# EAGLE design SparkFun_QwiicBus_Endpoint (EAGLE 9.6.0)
ABBREV: hb1; PROJECT: Heading Board
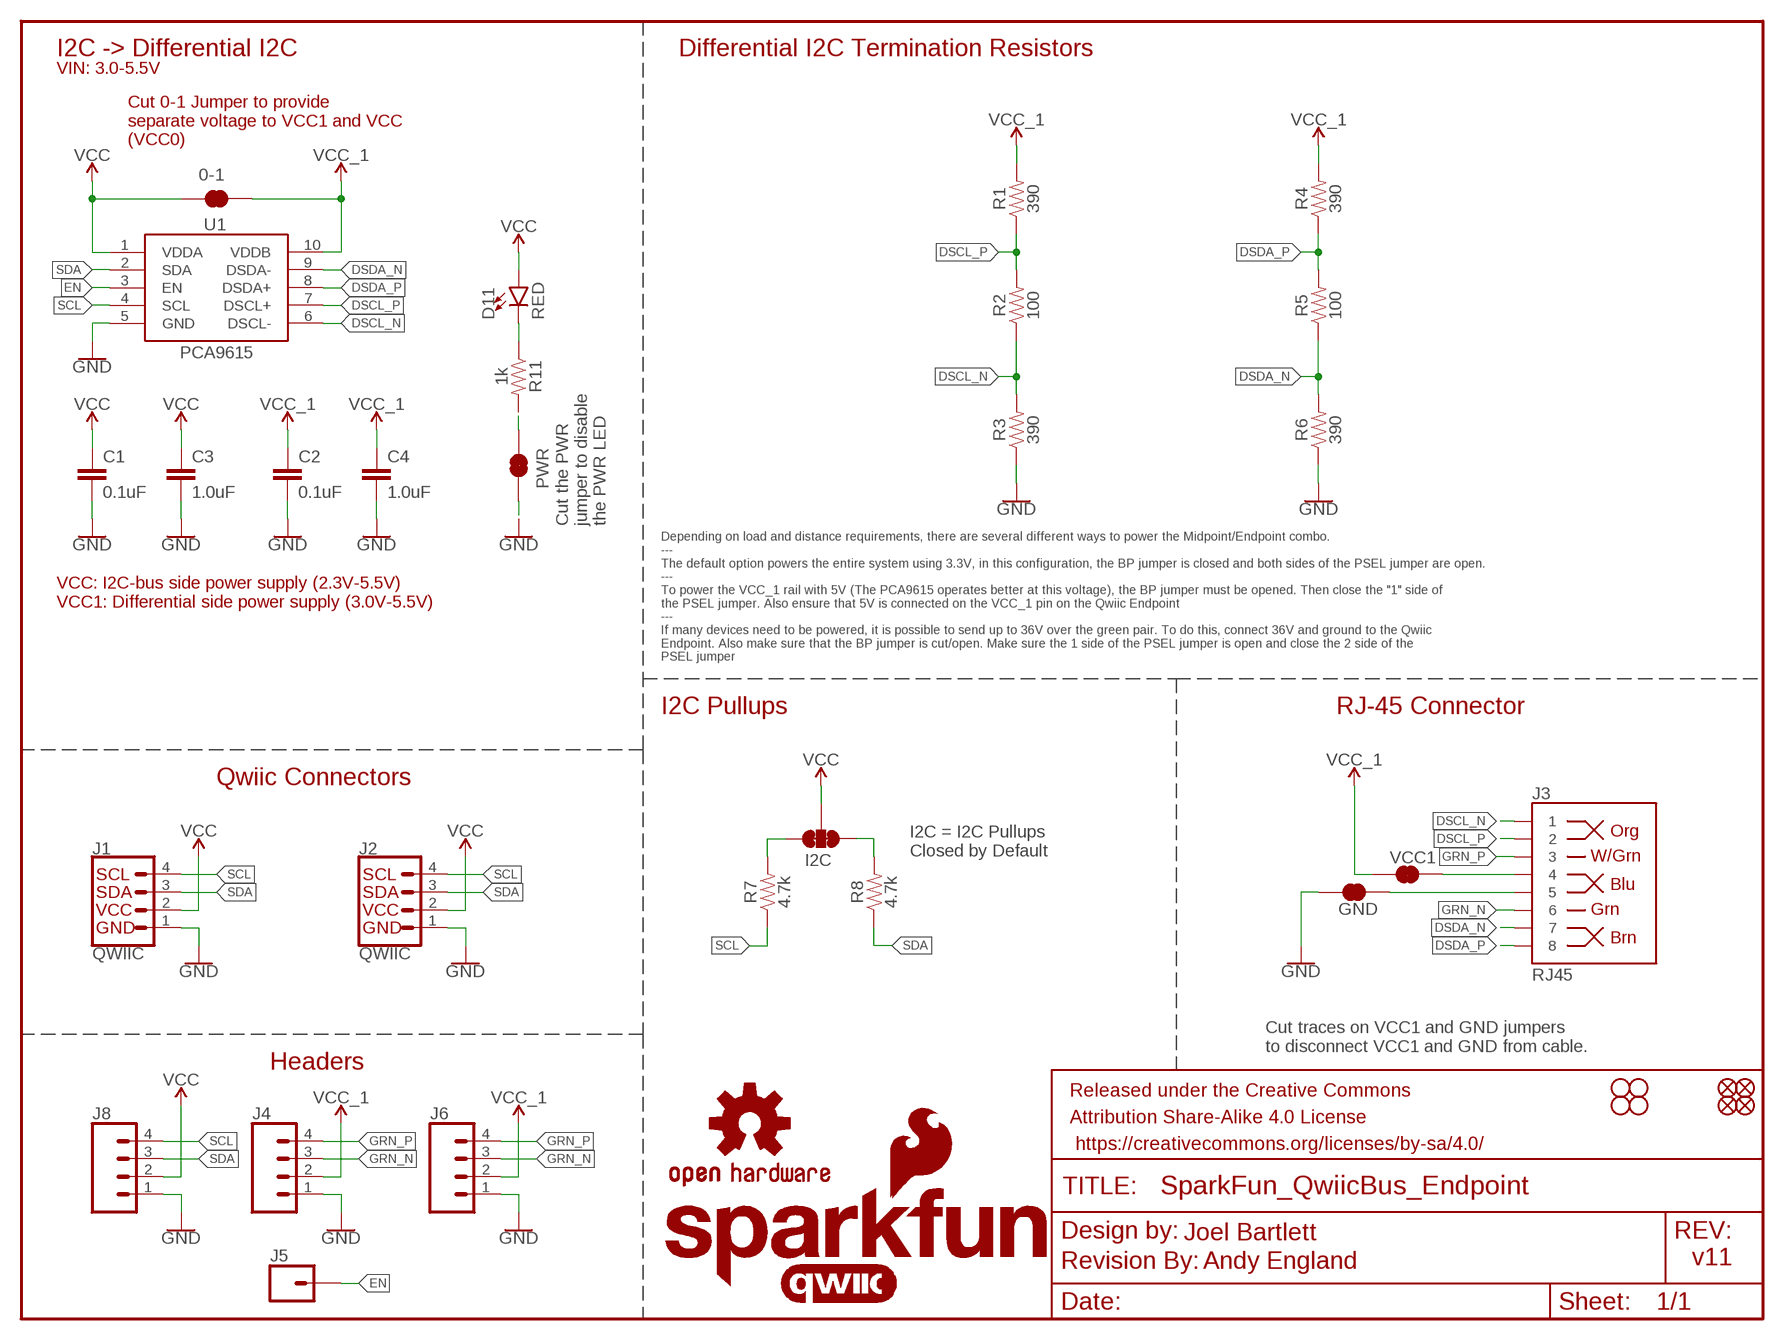
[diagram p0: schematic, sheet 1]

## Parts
0-1  JUMPER-SMT_2_NC_TRACE_SILK  [SMT-JUMPER_2_NC_TRACE_SILK]
C1  0.1uF  0.1UF-0603-25V-(+80/-20%)  [0603]
C2  0.1uF  0.1UF-0603-25V-(+80/-20%)  [0603]
C3  1.0uF  1.0UF-0603-16V-10%  [0603]
C4  1.0uF  1.0UF-0603-16V-10%  [0603]
D11  RED  LED-RED0603  [LED-0603]
FD1  FIDUCIALUFIDUCIAL  [FIDUCIAL-MICRO]
FD2  FIDUCIALUFIDUCIAL  [FIDUCIAL-MICRO]
FD3  FIDUCIALUFIDUCIAL  [FIDUCIAL-MICRO]
FD4  FIDUCIALUFIDUCIAL  [FIDUCIAL-MICRO]
FRAME1  FRAME-LETTER  [CREATIVE_COMMONS]
GND  JUMPER-SMT_2_NC_TRACE_SILK  [SMT-JUMPER_2_NC_TRACE_SILK]
H1  STAND-OFF  [STAND-OFF]
H2  STAND-OFF  [STAND-OFF]
H3  STAND-OFF  [STAND-OFF]
H4  STAND-OFF  [STAND-OFF]
I2C  JUMPER-SMT_3_2-NC_TRACE_SILK  [SMT-JUMPER_3_2-NC_TRACE_SILK]
J1  QWIIC  QWIIC_CONNECTORJS-1MM  [JST04_1MM_RA]
J2  QWIIC  QWIIC_CONNECTORJS-1MM  [JST04_1MM_RA]
J3  RJ45  RJ45-8  [RJ45-8]
J4  CONN_041X04_NO_SILK  [1X04_NO_SILK]
J5  CONN_01PTH_NO_SILK_YES_STOP  [1X01_NO_SILK]
J6  CONN_041X04_NO_SILK  [1X04_NO_SILK]
J8  CONN_041X04_NO_SILK  [1X04_NO_SILK]
LOGO1  OSHW-LOGOM  [OSHW-LOGO-M]
LOGO2  REVISION  [REVISION]
LOGO3  QWIIC_LOGO_4MM  [QWIIC_4MM]
LOGO4  SFE_LOGO_NAME_FLAME.1_INCH  [SFE_LOGO_NAME_FLAME_.1]
LOGO5  SFE_LOGO_FLAME.1_INCH  [SFE_LOGO_FLAME_.1]
PWR  JUMPER-SMT_2_NC_TRACE_SILK  [SMT-JUMPER_2_NC_TRACE_SILK]
R1  390  390OHM-0603-1/10W-1%  [0603]
R2  100  100OHM-0603-1/10W-1%  [0603]
R3  390  390OHM-0603-1/10W-1%  [0603]
R4  390  390OHM-0603-1/10W-1%  [0603]
R5  100  100OHM-0603-1/10W-1%  [0603]
R6  390  390OHM-0603-1/10W-1%  [0603]
R7  4.7k  4.7KOHM-0603-1/10W-1%  [0603]
R8  4.7k  4.7KOHM-0603-1/10W-1%  [0603]
R11  1k  1KOHM-0603-1/10W-1%  [0603]
U1  PCA9615  [TSSOP10]
VCC1  JUMPER-SMT_2_NC_TRACE_SILK  [SMT-JUMPER_2_NC_TRACE_SILK]

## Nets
DSCL_N: J3.1 R2.1 R3.2 U1.6(DSCL-)
DSCL_P: J3.2 R1.1 R2.2 U1.7(DSCL+)
DSDA_N: J3.7 R5.1 R6.2 U1.9(DSDA-)
DSDA_P: J3.8 R4.1 R5.2 U1.8(DSDA+)
EN: J5.1 U1.3(EN)
GND: C1.2 C2.2 C3.2 C4.2 GND.1 J1.1 J2.1 J4.1 J6.1 J8.1 PWR.1 R3.1 R6.1 U1.5(GND)
GRN_N: J3.6 J4.3 J6.3
GRN_P: J3.3 J4.4 J6.4
N$1: J3.4 VCC1.2
N$2: GND.2 J3.5
N$3: I2C.1 R8.2
N$4: I2C.3 R7.2
N$13: D11.C R11.1
N$14: PWR.2 R11.2
SCL: J1.4 J2.4 J8.4 R7.1 U1.4(SCL)
SDA: J1.3 J2.3 J8.3 R8.1 U1.2(SDA)
VCC: 0-1.2 C1.1 C3.1 D11.A I2C.2 J1.2 J2.2 J8.2 U1.1(VDDA)
VCC_1: 0-1.1 C2.1 C4.1 J4.2 J6.2 R1.2 R4.2 U1.10(VDDB) VCC1.1

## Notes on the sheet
- I2C -> Differential I2C | Differential I2C Termination Resistors
- VIN: 3.0-5.5V
- Cut 0-1 Jumper to provide
  separate voltage to VCC1 and VCC
  (VCC0)
- Cut the PWR 
  jumper to disable
  the PWR LED
- VCC: I2C-bus side power supply (2.3V-5.5V)
  VCC1: Differential side power supply (3.0V-5.5V)
- Depending on load and distance requirements, there are several different ways to power the Midpoint/Endpoint combo. 
  ---
  The default option powers the entire system using 3.3V, in this configuration, the BP jumper is closed and both sides of the PSEL jumper are open.
  ---
  To power the VCC_1 rail with 5V (The PCA9615 operates better at this voltage), the BP jumper must be opened. Then close the "1" side of 
  the PSEL jumper. Also ensure that 5V is connected on the VCC_1 pin on the Qwiic Endpoint
  ---
  If many devices need to be powered, it is possible to send up to 36V over the green pair. To do this, connect 36V and ground to the Qwiic 
  Endpoint. Also make sure that the BP jumper is cut/open. Make sure the 1 side of the PSEL jumper is open and close the 2 side of the
  PSEL jumper
- I2C Pullups | RJ-45 Connector
- Qwiic Connectors
- I2C = I2C Pullups
  Closed by Default
- Cut traces on VCC1 and GND jumpers 
  to disconnect VCC1 and GND from cable.
- Headers
- Joel Bartlett
- Andy England | v11

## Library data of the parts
0-1 GND PWR VCC1 = SparkFun-Jumpers:JUMPER-SMT_2_NC_TRACE: Normally closed trace jumper
C1 C2 = SparkFun-Capacitors:0.1UF: 0.1µF ceramic capacitors; PROD_ID: CAP-00810
C3 C4 = SparkFun-Capacitors:1.0UF: 1µF ceramic capacitors; PROD_ID: CAP-00868
D11 = SparkFun-LED:LED-RED: Red SMD LED; PROD_ID: DIO-00819
FD1-FD4 = SparkFun-Aesthetics:FIDUCIAL: Fiducial Alignment Points
FRAME1 = SparkFun-Aesthetics:FRAME-LETTER: Schematic Frame - Letter
H1-H4 = SparkFun-Hardware:STAND-OFF: Stand Off
I2C = SparkFun-Jumpers:JUMPER-SMT_3_2-NC_TRACE: Normally closed trace jumper (2 of 2 connections) This jumper has a trace between all three pads so they are normally closed (NC). Use a razor knife to open the connection(s). For best results follow the IPC guidelines for cutting traces: Cutout at least 0.063 mm (0.005 in). Remove all loose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
J1 J2 = SparkFun-Connectors:QWIIC_CONNECTOR: SparkFun I2C Standard Qwiic Connector An SMD 1mm pitch JST connector makes it easy and quick (get it? Qwiic?) to connect I2C devices to each other. The Qwiic system enables fast and solderless connection between popular platforms and various sensors and actuators. We carry 200mm, 100mm, 50mm, and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; PROD_ID: CONN-13694; VALUE: QWIIC_RIGHT_ANGLE
J3 = SparkFun-Connectors:RJ45-8: RJ45 Jack - 8 pin Simple RJ45, 8-pin connection. Commonly used for Cat5, Cat5e, and Cat6 Ethernet cables. Here is the connector we sell at SparkFun: RJ45 8-Pin Connector (PRT-00643) Datasheet It is used on this SparkFun product: SparkFun RJ45 Breakout (BOB-00716) Note, you may also be interested in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; PROD_ID: CONN-08506; SF_ID: PRT-00643
J4 J6 J8 = SparkFun-Connectors:CONN_04: Multi connection point. Often used as Generic Header-pin footprint for 0.1 inch spaced/style header connections On any of the 0.1 inch spaced packages, you can populate with these: Break Away Headers - Straight (PRT-00116) Break Away Male Headers - Right Angle (PRT-00553) Female Headers (PRT-00115)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; PROD_ID: CONN-09696
J5 = SparkFun-Connectors:CONN_01: Single connection point. Often used as Generic Header-pin footprint for 0.1 inch spaced/style header connections
LOGO1 = SparkFun-Aesthetics:OSHW-LOGO: Open-Source Hardware (OSHW) Logo
LOGO2 = SparkFun-Aesthetics:REVISION: "Revision By" Text
LOGO3 = SparkFun-Aesthetics:QWIIC_LOGO: Qwiic Logos for placement on schematic and PCB. The 5.5mm silk logo is best for placing next to Qwiic connector.
LOGO4 = SparkFun-Aesthetics:SFE_LOGO_NAME_FLAME: SparkFun Font Logo w/ Flame
LOGO5 = SparkFun-Aesthetics:SFE_LOGO_FLAME: SparkFun Flame Logo
R1 R3 R4 R6 = SparkFun-Resistors:390OHM: 390Ω resistor; PROD_ID: RES-07864
R2 R5 = SparkFun-Resistors:100OHM: 100Ω resistor; PROD_ID: RES-07863
R7 R8 = SparkFun-Resistors:4.7KOHM: 4.7kΩ resistor; PROD_ID: RES-07857
R11 = SparkFun-Resistors:1KOHM: 1kΩ resistor; PROD_ID: RES-07856
U1 = SparkFun-IC-Comms:PCA9615: Differential I2C Bus Buffer Datasheet; PROD_ID: IC-13899

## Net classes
0 default: width 0.203 mm
1 power: width 0.381 mm, clearance 0.254 mm

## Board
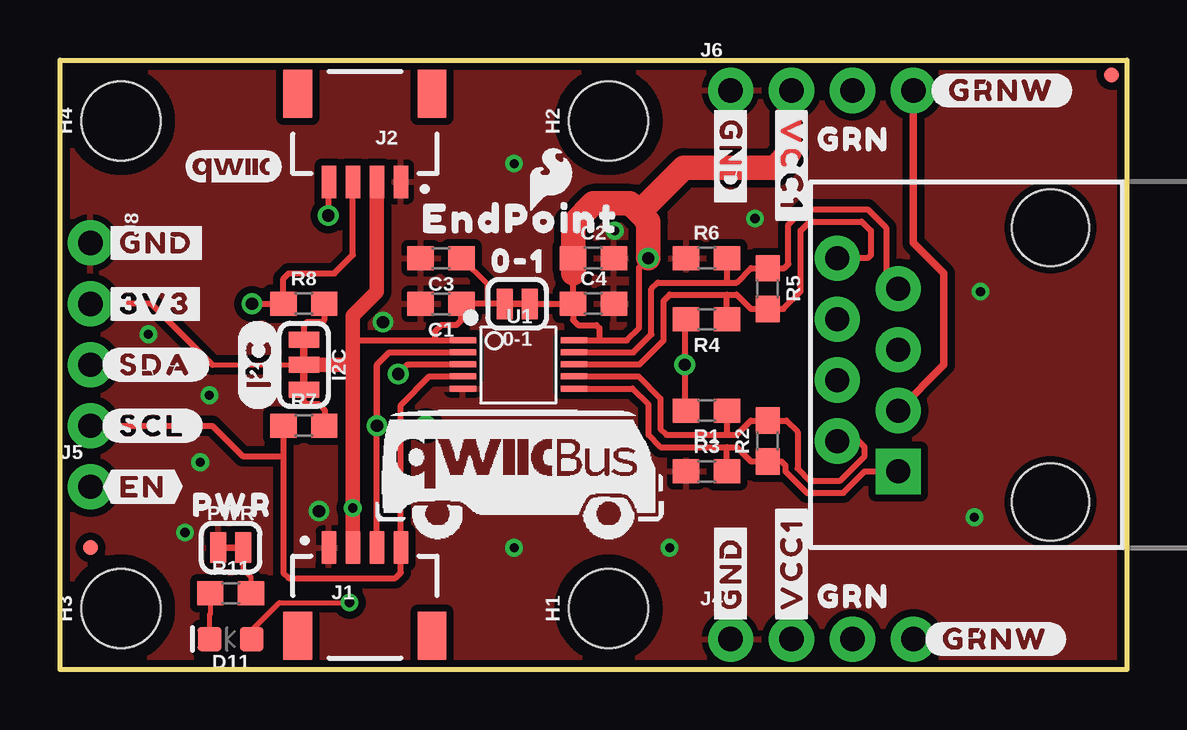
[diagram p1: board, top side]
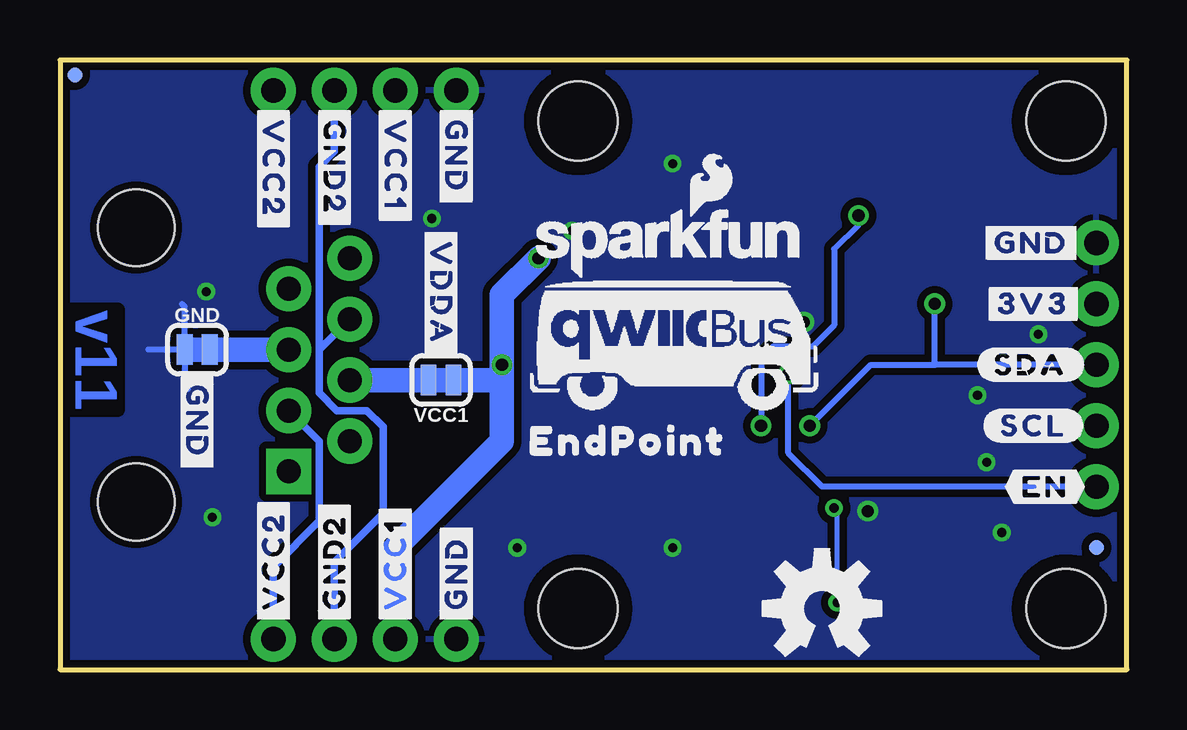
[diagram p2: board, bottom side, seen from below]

Size 44.45 x 25.4 mm. Coordinates in mm from the lower left corner, seen from the top.
Outline: 44.45,0 0,0 0,25.4 44.45,25.4 44.45,0
Copper layers (1*16): Top 0.035mm / dielectric 1.5mm / Bottom 0.035mm
Design rules "SparkFun-2-layer-TIGHT": minimum track width 7mil, minimum drill 15mil, track to track 7mil, track to pad 7mil, pad to pad 7mil, via to via 7mil, smd to smd 7mil, copper to edge 7mil, drill to drill 7mil, minimum pad ring 7mil, minimum via ring 7mil, stop-mask expansion 4mil, vias tented up to drill 25mil, thermal gap 10mil

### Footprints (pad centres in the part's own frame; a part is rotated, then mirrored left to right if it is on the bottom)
SMT-JUMPER_2_NC_TRACE_SILK = smd 0.66 x 1.27: 1 -0.521,0; 2 0.521,0
0603 = smd 1.1 x 1: 1 -0.85,0; 2 0.85,0
LED-0603 = smd 1 x 1: A -0.877,0; C 0.877,0
FIDUCIAL-MICRO = smd 0.635 x 0.635: 1 0,0
STAND-OFF = hole 3.302: 0,0
SMT-JUMPER_3_2-NC_TRACE_SILK = smd 0.66 x 1.27: 1 -1.041,0; 2 0,0; 3 1.041,0
JST04_1MM_RA = smd 0.6 x 1.35: 1 -1.5,0; 2 -0.5,0; 3 0.5,0; 4 1.5,0 | smd 1.2 x 2: NC1 2.8,-3.675; NC2 -2.8,-3.675
RJ45-8 = drill 1 pad 1.88 square: 1 -4.445,6.35 | drill 1 pad 1.88: 2 -3.175,8.89; 3 -1.905,6.35; 4 -0.635,8.89; 5 0.635,6.35; 6 1.905,8.89; 7 3.175,6.35; 8 4.445,8.89 | hole 3.2: -5.715,0; 5.715,0
1X04_NO_SILK = drill 1.016 pad 1.88: 1 0,0; 2 2.54,0; 3 5.08,0; 4 7.62,0
1X01_NO_SILK = drill 1.016 pad 1.88: 1 0,0
TSSOP10 = smd 1.1 x 0.25: 1 -2.259,1.018; 2 -2.259,0.517; 3 -2.259,0.018; 4 -2.259,-0.482; 5 -2.259,-0.988; 6 2.366,-0.988; 7 2.366,-0.482; 8 2.366,0.018; 9 2.366,0.517; 10 2.366,1.018

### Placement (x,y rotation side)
0-1  19.05,15.24 180 top
C1  15.88,15.24 180 top
C2  22.23,17.14 0 top
C3  15.88,17.14 180 top
C4  22.23,15.24 0 top
D11  7.11,1.27 180 top
FD1  1.27,5.08 0 top
FD2  43.81,24.77 0 top
FD3  1.27,5.08 0 bottom
FD4  43.81,24.77 0 bottom
FRAME1  not placed on the board
GND  38.73,13.34 0 bottom
H1  22.86,2.54 90 top
H2  22.86,22.86 90 top
H3  2.54,2.54 90 top
H4  2.54,22.86 90 top
I2C  10.16,12.7 270 top
J1  12.7,5.08 0 top
J2  12.7,20.32 180 top
J3  41.27,12.7 90 top
J4  27.94,1.27 0 top
J5  1.27,7.62 0 top
J6  27.94,24.13 0 top
J8  1.27,17.78 270 top
LOGO1  12.7,2.54 0 bottom
LOGO2  not placed on the board
LOGO3  7.24,20.95 0 top
LOGO4  19.05,17.78 0 bottom
LOGO5  20.45,20.45 0 top
PWR  7.11,5.08 0 top
R1  26.94,10.79 180 top
R2  29.48,9.53 90 top
R3  26.94,8.26 0 top
R4  26.94,14.61 180 top
R5  29.48,15.88 270 top
R6  26.94,17.14 0 top
R7  10.16,10.16 0 top
R8  10.16,15.24 0 top
R11  7.11,3.17 0 top
U1  19.05,12.7 0 top
U$1  [I2C]  8.26,10.79 90 top
U$2  [GRN0]  30.86,3.05 0 top
U$3  [#GND#0]  27.94,1.78 90 top
U$4  [#GND#0]  6.22,17.78 0 bottom
U$5  [#GND#0]  1.78,17.78 0 top
U$6  [#GND#0]  38.73,12.57 270 bottom
U$7  [#3V3#0]  1.78,15.24 0 top
U$8  [#3V3#0]  6.1,15.24 0 bottom
U$9  [#SDA#0]  1.78,12.7 0 top
U$10  [#SCL#0]  1.78,10.16 0 top
U$11  [#EN#0]  1.78,7.62 0 top
U$12  [#VDDA#0]  28.57,18.54 270 bottom
U$13  [#GND#0]  27.94,1.78 90 bottom
U$14  [#GND2#0]  33.02,23.62 270 bottom
U$15  [#SDA#0]  6.22,12.7 0 bottom
U$16  [#SCL#0]  5.97,10.16 0 bottom
U$17  [#EN#0]  5.08,7.62 0 bottom
U$18  [#GND2#0]  33.02,1.78 90 bottom
U$19  [#GRNW#0]  36.07,1.27 0 top
U$20  [#VCC1#0]  30.48,1.78 90 top
U$21  [#VCC1#0]  30.48,1.78 90 bottom
U$22  [#GRNW#0]  36.32,24.13 0 top
U$23  [QWIICBUS#WORKING#LOGO#JPG]  18.44,13.87 0 bottom
U$24  [#VCC2#0]  35.56,1.78 90 bottom
U$25  [0#10]  17.27,17.02 0 top
U$26  [ENDPOINT0]  25.78,9.53 0 bottom
U$27  [PWR0]  4.83,6.86 0 top
U$28  [QWIICBUS#WORKING#LOGO#JPG]  19.56,8.51 0 top
U$29  [GRN0]  30.86,22.1 0 top
U$30  [#VCC2#0]  35.56,23.62 270 bottom
U$31  [#VCC1#0]  30.48,23.62 270 bottom
U$32  [#VCC1#0]  30.48,23.62 270 top
U$33  [#GND#0]  27.94,23.62 270 bottom
U$34  [#GND#0]  27.94,23.62 270 top
U$35  [ENDPOINT0]  14.22,18.8 0 top
VCC1  28.57,12.06 180 bottom

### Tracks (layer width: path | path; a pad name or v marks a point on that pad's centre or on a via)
DSCL_N
  Top 0.254: U1.6 23.85,11.71 24.51,11.05 24.51,9.78 25.02,9.27 27.79,9.27 | R3.2 27.79,9.27 | J3.1 33.53,8.26 32.64,7.37 31.11,7.37 30.23,8.26 30.23,8.51 30.06,8.68 R2.1 28.79,8.68 28.19,9.27 27.79,9.27
DSCL_P
  Top 0.254: U1.7 24.11,12.22 25.02,11.3 25.02,10.03 25.27,9.78 27.79,9.78 | R1.1 27.79,9.78 | J3.2 33.27,9.53 33.53,9.27 33.53,8.89 32.51,7.87 31.24,7.87 30.73,8.38 30.73,9.91 30.27,10.38 R2.2 28.79,10.38 28.19,9.78 27.79,9.78
DSDA_N
  Top 0.254: U1.9 23.89,13.22 24.64,13.97 24.64,15.86 24.91,16.13 27.79,16.13 | R6.2 27.79,16.13 | J3.7 34.42,16.38 34.42,18.41 33.66,19.18 30.99,19.18 30.35,18.54 30.35,16.89 30.19,16.73 R5.1 28.79,16.73 28.19,16.13 27.79,16.13
DSDA_P
  Top 0.254: J3.8 33.66,17.14 33.78,17.27 33.78,18.29 33.4,18.67 31.24,18.67 30.86,18.29 30.86,15.75 30.14,15.03 R5.2 28.79,15.03 28.19,15.62 27.79,15.62 | U1.8 24.15,12.72 25.15,13.72 25.15,15.37 25.4,15.62 27.79,15.62 | R4.1 27.79,15.62
EN  (via drill 0.51)
  Top 0.254: U1.3 14.49,12.72 v14.1,12.32
  Bottom 0.254: J5.1 12.7,7.62 14.1,9.02 v14.1,12.32
GND  (via drill 0.38, 0.51)
  Bottom 0.254: GND.1 39.26,15.13 39.37,15.24 | GND.1 40.77,13.34 | GND.1 39.26,11.82 39.12,11.68
  other vias: 10.79,6.6 5.21,5.71 13.46,14.48 23.11,18.29 38.35,15.75 5.84,8.64 6.22,11.43 3.68,13.97 18.92,5.08 18.92,21.08 28.96,18.8 25.4,5.08 38.1,6.35
  pour Top (isolate 0.305): 44.45,0 0,0 0,25.4 44.45,25.4
  pour Bottom (isolate 0.305): 44.45,0 0,0 0,25.4 44.45,25.4
GRN_N
  Bottom 0.305: 33.66,13.34 33.66,11.54 32.91,10.79 31.67,10.79 30.99,10.12 30.99,6.51 33.02,4.48 J4.3 | J3.6 33.66,13.34 | 33.66,13.34 33.66,20.95 33.02,21.59 J6.3
GRN_P
  Top 0.305: J6.4 35.56,17.78 36.83,16.51 36.83,12.7 J3.3
  Bottom 0.305: J3.3 33.66,9.53 33.66,6.21 33.64,6.19 35.56,4.27 J4.4
N$1
  Bottom 1.016: J3.4 VCC1.2 28.07,12.06
N$2
  Bottom 1.016: J3.5 GND.2 39.12,13.34
N$3
  Top 0.254: R8.2 11.01,14.57 10.92,14.48 10.29,14.48 10.16,14.35 I2C.1
N$4
  Top 0.254: R7.2 11.05,10.2 11.05,10.79 10.79,11.05 10.29,11.05 10.16,11.18 I2C.3
N$13
  Top 0.203: R11.1 6.26,2.33 6.22,2.29 6.22,1.28 D11.C
N$14
  Top 0.203: R11.2 7.96,3.85 7.63,4.18 PWR.2
SCL  (via drill 0.51)
  Top 0.254: R7.1 9.31,8.89 | 9.31,8.89 9.31,4.03 9.53,3.81 13.97,3.81 14.2,4.04 J1.4 14.2,10.16 | 14.2,10.16 14.2,11.03 15.39,12.22 U1.4 | v15.24,10.16 14.2,10.16 | v11.18,18.92 11.2,18.95 J2.4 | J8.4 6.35,10.16 7.62,8.89 9.31,8.89
  Bottom 0.254: v15.24,10.16 15.24,12.95 14.73,13.46 13.08,13.46 12.19,14.35 12.19,17.53 11.18,18.54 v11.18,18.92
SDA  (via drill 0.51)
  Top 0.254: v8,15.24 R8.1 9.31,16.3 9.53,16.51 11.43,16.51 12.2,17.28 J2.3 | J1.3 13.2,12.69 13.21,12.7 | U1.2 13.73,13.22 13.21,12.7 | 13.21,12.7 v13.21,10.16
  Bottom 0.254: v13.21,10.16 10.67,12.7 8,12.7 | 8,12.7 v8,15.24 | J8.3 8,12.7
VCC  (via drill 0.38)
  Top 0.203: D11.A 7.99,1.64 9.14,2.79 v12.06,2.79 | C3.1 17.78,16.09 17.78,15.24 | 6.35,12.7 I2C.2
  Top 0.254: U1.1 15.62,13.72 | 6.35,12.7 3.81,15.24 J8.2 | 0-1.2 17.78,15.24 C1.1 16.73,14.57 16.64,14.48 16.51,14.35 15.88,14.35 15.62,14.1 15.62,13.72 | 12.2,13.97 12.45,13.72 15.62,13.72
  Top 0.61: J2.2 13.2,15.74 12.2,14.74 12.2,13.97 12.2,12.7 | 12.2,12.7 v12.2,6.73 J1.2 | I2C.2 12.2,12.7
  Bottom 0.203: v12.06,2.79 12.06,6.6 v12.2,6.73
VCC_1  (via drill 0.51)
  Top 0.254: 22.48,13.72 22.48,14.22 22.35,14.35 21.59,14.35 21.38,14.57 C4.1 | 22.48,13.72 23.62,13.72 24.13,14.22 24.13,16.76 v24.51,17.14 | 21.33,18.63 21.38,18.58 | 0-1.1 C4.1 | C4.1 21.38,16.51 C2.1 | R1.2 26.04,10.85 v26.04,12.7 26.04,14.55 R4.2 | U1.10 22.48,13.72
  Top 1.016: v24.51,17.14 24.51,18.67 24.13,19.05 | 24.13,19.05 23.75,19.43 22.23,19.43 21.38,18.58 21.38,16.51 | 24.13,19.05 26,20.92 29.77,20.92 30.39,21.53 30.39,24.04 J6.2
  Bottom 1.016: v24.51,17.14 26.04,15.62 v26.04,12.7 26.04,12.19 | J4.2 30.48,5.08 26.04,9.53 26.04,12.19 | 26.04,12.19 26.16,12.06 VCC1.1

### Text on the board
Bottom: v11
tDocu: Joel Bartlett | Andy England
